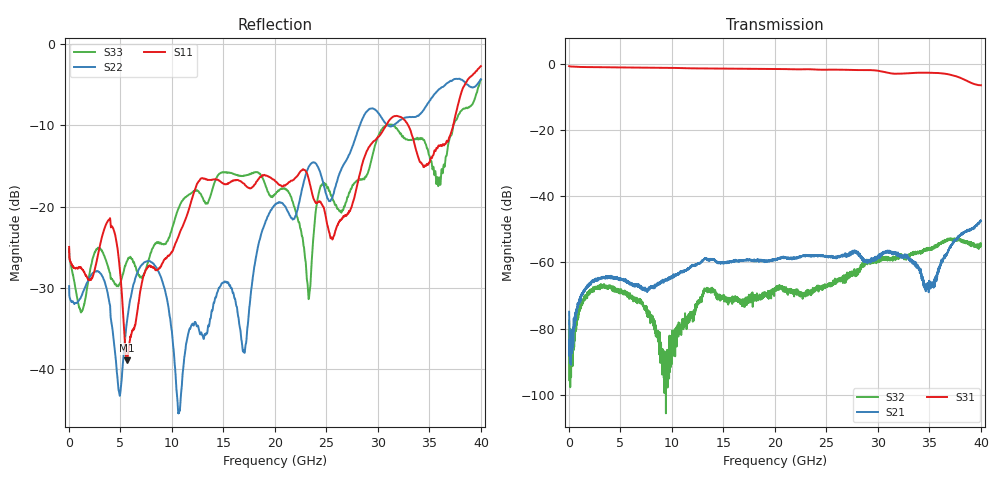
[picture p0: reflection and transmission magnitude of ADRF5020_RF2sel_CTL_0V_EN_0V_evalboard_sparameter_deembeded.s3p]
! Device:  ADRF5020
! Description: SOI MMIC SPDT Non-Reflective Switch
! Frequency:  0.1 -  30 GHz
! Ports:
! 	RFC	= Port 1
!	RF1	= Port 2
!	RF2	= Port 3
! Vdd:  +3.3 Volt
! Vss:  -2.5 Volt
! Control:  0/+3.3 Volt
! State:  RF2 Selected (Vctl= 0 V, Ven= 0 V)
! Data:	Data was collected using a calibrated network analyzer with AFR software.
!	Fixtures were calculated using AFR and fixturing was applied to collect
!	this Deembedded  S Parameter data of ADRF5020.
! Note:	Analog Devices supplies this data as a sample of measured data at the package pin
!	for this product.  Your particular data for this product may vary.
!	Data was taken at 25 degrees C.
!	Analog Devices reserves the right to change this data at anytime.
# Hz S  dB  R 50
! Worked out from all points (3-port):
!   4000 points, 10 MHz to 40 GHz, reference 50 ohm
!   strongest paths, dB at 10 MHz, 10.01 GHz, 20.01 GHz, 30.01 GHz, 40 GHz:
!     S31: -0.7, -1.2, -1.5, -2.0, -6.4
!     S21: -74.9, -64.4, -59.1, -58.2, -47.4
!     S32: -77.6, -84.5, -68.3, -59.0, -54.2
!   lowest |S11| = -38.9 dB at 5.62 GHz (marker M1), VSWR 1.02, Z = 48.9 - j0.288 ohm
!   |S11| at or under -10 dB: start of sweep to 30.8 GHz; 32.94 GHz to 37.32 GHz (4.386 GHz wide, 12.5 % of centre)
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1e7  -24.97 -6.2  -80.02 -167.2  -0.67 -0.5
     -74.90 24.7  -29.79 148.2  -81.49 65.8
     -0.67 -0.4  -77.61 162.8  -25.27 -4.7
4.04e9  -22.33 -81.1  -64.54 50.5  -1.02 -49.4
        -64.40 49.7  -33.56 -160.2  -67.84 12.4
        -1.01 -49.4  -67.17 16.6  -28.87 -131.8
5.62e9  -38.91 -165.0  -65.79 49.1  -1.07 -68.5
        -65.64 48.5  -34.22 117.8  -69.93 -6.2
        -1.06 -68.4  -69.69 -2.8  -26.75 -90.9
1.032e10  -24.57 -70.2  -64.16 108.0  -1.20 -125.3
          -63.91 105.6  -40.20 -58.0  -81.14 128.0
          -1.20 -125.1  -83.30 159.1  -21.41 -86.2
1.349e10  -16.72 -89.2  -59.30 95.4  -1.34 -164.3
          -59.18 95.1  -34.81 -55.7  -68.77 75.9
          -1.34 -164.1  -68.21 69.1  -19.56 -79.4
2.001e10  -16.85 -154.9  -59.10 87.0  -1.49 115.5
          -59.11 86.6  -19.79 -29.4  -67.77 -58.6
          -1.49 115.7  -68.26 -56.7  -18.46 -155.0
2.329e10  -16.69 -97.0  -58.01 72.3  -1.59 73.5
          -57.96 73.1  -15.09 -40.9  -69.47 -118.5
          -1.59 73.8  -69.35 -120.3  -31.35 -159.3
2.895e10  -13.12 -128.4  -60.08 26.9  -1.85 -1.7
          -59.65 27.6  -8.25 -72.8  -60.22 144.2
          -1.85 -1.4  -60.04 149.7  -16.03 -100.2
3.476e10  -14.75 -145.0  -67.05 27.1  -2.65 -87.0
          -66.62 24.1  -7.49 -105.7  -55.82 32.1
          -2.65 -86.6  -55.93 31.9  -12.85 -116.4
4e10  -2.72 -125.8  -47.45 47.5  -6.43 -174.4
      -47.39 49.1  -4.33 -117.9  -54.65 -102.1
      -6.43 -174.0  -54.23 -98.2  -4.39 -90.2
